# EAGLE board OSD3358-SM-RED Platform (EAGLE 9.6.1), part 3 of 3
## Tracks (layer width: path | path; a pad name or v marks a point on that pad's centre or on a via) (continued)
PMIC_PGOOD  (via drill 0.3) (continued)
  Bottom 0.152: v56.92,32.79 56.92,33.22 57.4,33.71 57.4,34.21 57.15,34.47 56.08,34.47 55.91,34.65 v55.91,35.38
PWR_BUT  (via drill 0.3)
  Top 0.152: U1.T11 57.4,35.46 v56.97,35.89 56.97,36.25 57.61,36.88 57.61,41.76 56.57,42.8 53.31,42.8 50.88,45.24 43.51,45.24 42.75,44.48 38.43,44.48 38,44.91 38,46.79 37.29,47.5 33.43,47.5 32.28,48.64 28.27,48.64 25.15,51.77 v24.18,51.77 | S2.4 12.43,51.37 12.5,51.44 | 12.5,51.44 v12.65,51.59 12.8,51.44 | S2.2 12.87,51.37 12.8,51.44 | 12.5,51.44 12.8,51.44
  Bottom 0.152: v56.97,35.89 56.44,36.42 55.68,36.42 54.56,35.31 53.09,35.31 50.95,33.17 50.95,32.89 50.57,32.51 50.57,25.04 48.54,23.01 48.54,14.58 51,12.12 51,5.56 50.37,4.93 50.37,2.97 J6.9 | v12.65,51.59 12.83,51.77 v24.18,51.77
PWR_EN  (via drill 0.3)
  Top 0.152: U1.N10 U1.N11 57.4,30.89 57.91,31.39 v57.91,31.5
  Bottom 0.152: v57.91,31.5 57.91,31.65 57.81,31.75 57.12,31.75 TP21.TP
RBIAS
  Top 0.152: U9.7 29.5,32.05 29.21,32.33 29.21,33.02 29.01,33.22 28.22,33.22 27.53,33.91 26.34,33.91 R115.1
RX_CLK
  Top 0.152: R94.1 R127.1 36.98,26.85 36.42,27.41 U9.31
RX_DV
  Top 0.152: U9.30 31.9,26.42 32.03,26.29 36.65,26.29 37.59,25.35 38.38,25.35 38.63,25.09 R101.1 R126.1
RXD0
  Top 0.152: R109.2 R125.1 36.6,25.15 35.76,25.98 31.9,25.98 31.5,26.39 U9.29
RXD1
  Top 0.152: U9.28 31.1,26.36 31.77,25.68 34.01,25.68 34.57,25.12 R106.2 R122.1
RXD2
  Top 0.152: R121.1 R98.1 32.54,25.15 32.31,25.38 30.43,25.38 30.12,25.68 30.12,26.16 30.3,26.34 U9.26
RXD3
  Top 0.152: R120.1 R95.1 30.18,24.82 30,24.99 30,25.38 29.82,25.55 29.82,26.42 29.9,26.49 U9.25
  Top 0.203: U9.25
SPI0_CS0
  Top 0.152: U18.C2 37.97,14.35 TP30.TP U21.1 39.8,14.69 39.57,14.91 R158.1
SPI0_D0(MISO)
  Top 0.152: U19.C2 38.76,12.61 TP29.TP U21.2
SPI0_D1(MOSI)
  Top 0.152: U20.C2 46.99,10.54 TP28.TP U21.5
SPI0_SCLK
  Top 0.152: U24.C2 46.33,12.41 TP27.TP U21.6
SPI1_CS0  (via drill 0.3)
  Top 0.152: U1.B1 71.32,16.89 71.6,16.61 v71.6,15.7 71.6,14.73 72.34,13.99 72.34,10.34 73.69,8.99 75.13,8.99 75.74,8.38 75.74,6.1 76.35,5.49 v77.57,5.49 | v78.72,19.43 78.72,19.81 79.5,20.6 82.53,20.6 84.73,22.81 84.73,28.19 86.72,30.18 87.96,30.18 90.55,32.76 U10.25
  Bottom 0.152: v71.6,15.7 71.96,15.7 72.26,16 77.95,16 78.72,16.76 v78.72,19.43 | J6.28 75.34,5.49 v77.57,5.49
SPI1_D0  (via drill 0.3)
  Top 0.152: v68.4,16.26 68.4,16.05 U1.A2 69.22,15.24 69.8,15.24 71.42,13.61 71.42,9.96 72.85,8.53 72.85,6.1 73.46,5.49 74.98,5.49 75.44,5.03 75.44,3.3 J6.29 | v77.95,19.43 77.95,19.76 79.1,20.9 82.4,20.9 84.43,22.94 84.43,28.32 86.59,30.48 87.83,30.48 90.05,32.69 U10.24
  Bottom 0.152: v68.4,16.26 68.1,16.56 67.67,16.56 67.41,16.31 67.41,15.93 67.79,15.54 69.6,15.54 70.36,16.31 77.83,16.31 78.41,16.89 78.41,18.47 77.95,18.92 v77.95,19.43
SPI1_D1
  Top 0.152: U1.B2 69.37,16.89 70,16.26 70.43,16.26 70.66,16.03 70.66,15.24 72.03,13.87 72.03,10.21 73.56,8.69 74.84,8.69 75.44,8.09 75.44,5.94 76.83,4.55 J6.30
SPI1_SCLK  (via drill 0.3)
  Top 0.152: v69.24,16.26 69.24,15.93 69.55,15.62 U1.A1 70.1,15.37 71.73,13.74 71.73,10.08 73.15,8.66 73.15,6.25 73.61,5.79 75.13,5.79 75.74,5.18 75.74,3.66 76.35,3.05 78.23,3.05 J6.31 | v77.19,19.43 77.19,19.74 78.66,21.21 82.27,21.21 84.12,23.06 84.12,28.45 86.46,30.79 87.68,30.79 89.55,32.65 U10.23
  Bottom 0.152: v69.24,16.26 69.6,16.61 77.7,16.61 78.11,17.02 78.11,18.06 77.19,18.97 v77.19,19.43
SYS_ADC_1P8V  (via drill 0.3)
  Top 0.152: U1.A7 62.1,15.24 62.1,13.39 v62.53,12.95 | v60.81,12.22 59.49,10.9 v57.38,10.9
  Bottom 0.152: R33.2 C10.1 57.15,11.12 v57.38,10.9 | v60.81,12.22 61.8,12.22 v62.53,12.95 63.78,14.2 72.29,14.2 72.87,14.78 73.84,14.78 74.68,13.95 74.68,12.95 79.17,8.46 79.17,4.65 J6.32
SYS_RESETN  (via drill 0.3)
  Top 0.152: U16.17 85.47,12.57 85.95,13.06 85.95,13.72 86.26,14.02 v88.24,14.02 | U1.R11 57.4,33.78 57.25,33.93 v56.74,33.93 56.19,33.93 55.37,34.75 55.37,35.69 55.93,36.25 v55.93,37.26 55.93,37.92 55.35,38.51 54.91,38.51 C94.1 R5.2 53.39,38.48 52.96,38.48 52.83,38.35 52.83,37.59 | v94.18,26.59 C14.1 95.38,26.59 95.5,26.72 95.5,29.08 95.68,29.26 96.55,29.26 96.62,29.34 97.16,29.34 97.28,29.21 101.6,29.21 102.23,29.84 J4.15 | v88.34,18.87 88.34,19.74 86.67,21.41 v86.67,22.94 | 6.44,52.95 7.53,52.95 8.18,52.3 8.18,50.93 8.61,50.49 v11.89,50.49 | v23.37,51.21 25.2,51.21 28.09,48.31 32.13,48.31 33.25,47.19 37.13,47.19 37.69,46.63 37.69,44.58 38.1,44.17 42.88,44.17 43.61,44.91 50.7,44.91 53.19,42.42 U3.4 53.19,41.76 52.88,41.45 52.5,41.45 51.82,40.77 51.82,38.48 51.36,38.02 51.36,37.54 51.69,37.21 52.45,37.21 52.7,37.47 | 52.7,37.47 52.83,37.59 | 52.83,37.59 52.96,37.47 | 52.96,37.47 53.75,36.68 TP26.P$1 | 52.7,37.47 52.96,37.47
  Top 0.254: S1.3 6.42,52.97 6.44,52.95 6.47,52.97 S1.1
  Bottom 0.152: J6.10 51.31,4.57 51.31,12.24 48.84,14.71 48.84,22.89 50.88,24.92 50.88,32.38 51.26,32.77 51.26,33.05 53.21,35 55.12,35 56.19,33.93 v56.74,33.93 | v88.24,14.02 88.24,18.77 v88.34,18.87 | v86.67,22.94 86.89,22.71 88.01,22.71 88.7,23.39 90.09,23.39 90.5,23.8 90.5,25.88 92.25,27.64 93.5,27.64 93.7,27.43 93.7,26.85 93.95,26.59 v94.18,26.59 94.74,27.15 94.74,30.2 94,30.94 91.01,30.94 90.4,31.55 86.77,31.55 84.76,29.54 83.19,29.54 83.03,29.39 83.03,28.07 82.83,27.86 80.95,27.86 80.72,28.09 77.39,28.09 76.71,28.78 76.71,30.81 76.2,31.32 74.3,31.32 71.4,28.42 69.52,28.42 69.14,28.04 67.44,28.04 66.52,28.96 64.47,28.96 63.7,29.72 63.7,32.69 62.08,34.31 58.6,34.31 57.81,35.1 57.81,36.25 56.97,37.08 56.11,37.08 v55.93,37.26 | v23.37,51.21 23.14,51.44 13.31,51.44 12.37,50.49 v11.89,50.49
SYS_RTC_1P8V  (via drill 0.3, 0.3 pad 0.61)
  Top 0.152: v52.07,37.8 52.32,38.05 52.32,39.88 TP14.TP 52.5,40.19 U3.5
  Bottom 0.152: U5.3 58.04,27 57.96,26.92 R15.1 | v56.9,27.69 57.95,27.69 U5.3 | U5.3 57.99,27.65 57.99,30.63 58.45,31.09 60.12,31.09 60.3,31.27 60.3,33.48 59.77,34.01 58.47,34.01 57.51,34.98 57.51,36.12 56.9,36.73 55.55,36.73 54.43,35.61 52.96,35.61 52.07,36.5 v52.07,37.8
  pour Top (rank 4): 56.77,26.54 56.77,28.96 58.04,28.96 58.04,26.42 56.77,26.42
  pour Bottom (no thermals): 57.63,26.14 60.17,26.14 60.38,26.34 60.38,27.97 60.2,28.14 57.66,28.14 57.48,27.97 56.77,27.97 56.64,27.84 56.64,27.28 56.87,27.05 57.23,27.05 57.48,26.8 57.48,26.29
SYS_VDD1_3P3V  (via drill 0.3, 0.3 pad 0.61, 0.5)
  Top 0.127: U7.M4 U7.N4 U7.P3 | U7.P5 77.54,40.54 v77.88,40.54 | U7.C6 U7.C7 U7.B8 U7.A9
  Top 0.152: C48.1 v19.68,11.43 R8.2 | R137.1 v33.07,12.95 | R96.1 v27.46,22.94 | R98.2 v32.54,22.94 | U16.1 80.78,15.74 80.64,15.88 v80.01,15.88 | C86.1 v91.19,12.45 | U17.D3 92.13,15.87 92.54,16.28 v93.09,16.28 | U16.8 v80.04,12.57 v80.03,12.57 | R13.2 v79.83,17.14 | 73.01,41.59 v73.13,41.71 | R44.2 R45.2 v53.37,44.93 | v57.45,45.7 R49.2 R48.2 | R130.2 v96.5,48.36 | C15.1 99.72,33.98 99.49,33.76 v99.49,33.4 | R12.2 v84.71,17.14 | R41.2 v94.18,25.53 | R144.2 v24.41,22.94 | R94.2 v39.88,25.83 | v30.5,22.94 R95.2 R93.2 | R145.1 v39.88,34.98 | Y5.4 74.13,15.76 73.89,16 72.59,16 72.49,16.1 72.49,16.94 v72.29,17.14 | R160.1 44.4,15.34 43.56,14.5 v42.55,14.5 | v37.47,16.13 37.72,15.88 U18.A2 | v37.47,13.08 37.72,12.83 U19.A2 | v47.5,8.76 47.25,9.01 U20.A2 | v47.5,11.81 47.25,12.06 U24.A2 | v38.48,9.73 39.04,9.73 39.24,9.53 R157.1 | R161.1 v37.47,8 | C85.1 86.67,14.63 v85.95,14.63 85.89,14.57 U16.22 | R40.2 v94.18,24.46 | R140.1 95.66,23.39 95.5,23.24 v95.5,22.73 | v92.2,29.84 91.39,29.84 Y3.4 | R158.2 v40.69,15.04 | U23.13 89.97,26.25 v89.97,25.2 | R5.1 53.11,39.8 52.88,39.57 v52.88,39.04 | U7.P2 U7.P1 76.99,39.12 | v69.47,43.08 69.48,43.09 U7.A9 | C87.1 v79.12,16.26
  Top 0.203: U9.3 31.1,32.12 31.47,32.49 32.18,32.49 32.64,32.94 32.64,33.5 32.84,33.71 R146.1 v33.25,32.99
  Top 0.254: U8.10 23.65,8.03 23.52,7.9 v22.91,7.9 | U8.29 27.15,14.78 27.58,15.21 v28.55,15.21 | U7.K9 74.51,43.09 | 74.51,43.09 74.49,43.09 U7.J10 | 74.51,43.09 v74.37,42.95 | U7.E6 73.01,41.59 | U7.F5 72.99,41.57 v73.13,41.71 | J4.5 v102.31,23.5 | R110.2 C39.1 v93.12,25.91 | v77.88,39.01 77.09,39.01 76.99,39.12 U7.P3 | v82.78,25.48 82.58,25.28 U22.1 82.15,25.03 U22.10 | C92.1 79.35,25.55 v79.88,25.55 79.93,25.55 80.16,25.78 U22.6
  Top 0.305: C51.1 v19.81,6.22 | U8.23 v29.72,11.43 | C93.1 v41.99,15.04 | C62.1 v22.48,8.64 | v46.35,14.35 U21.8 | v105.49,11.3 C22.1 R90.2 R89.2 R88.2 R87.2 R91.2 R86.2 v105.54,17.4 | C21.1 95.25,19.81 v93.85,19.81 | U8.15 26.15,7.25 v26.67,6.73 | C79.1 C88.1 78.66,11.68 v79.5,11.68
  Top 0.381: C63.1 v30,15.65
  Bottom 0.152: C6.2 | R84.2 R85.2 | R52.2 77.6,35.92 77.29,35.61 v76.96,35.61 | R22.2 53.87,27.79 54.13,27.53 v54.28,27.53 | C43.1 72.54,17.4 v72.29,17.14 | R92.2 v89.46,12.5 | R17.2 88.67,25.2 v89.97,25.2 | TP12.TP 62.13,22.61 v63.12,22.61
  Bottom 0.203: R146.1 v33.25,32.99
  Bottom 0.254: U6.7 U6.8 67.91,11.49 v67.56,11.15 | C6.2 v74.98,11.79 | v66.02,45.61 R46.2 R47.2 | R43.2 R42.2 v68,45.68 | R78.2 v87.61,45.54 | R79.2 v88.67,45.54 | R85.2 v95.07,45.54 | R83.2 R82.2 v91.87,45.54 | R81.2 v90.81,45.54 | R80.2 v89.74,45.54 | R76.2 R75.2 R73.2 R74.2 | R76.2 v85.47,45.54 | R77.2 R76.2 | R72.2 R71.2 R70.2 81.51,45.82 v80.37,45.82 | C20.2 C18.2 C19.2 v75.06,46.43 | R51.2 R50.2 69.98,45.68 v69.88,45.58 | C17.2 75.34,42.95 v74.37,42.95 | C90.2 89.69,23.95 89.97,24.23 v89.97,25.2
  Bottom 0.305: C16.2 v65.66,41.05 | X3.4 91.77,19.81 v93.85,19.81 | R143.2 22.55,15.67 22.99,15.24 v22.99,14.1 | v29.72,11.43 29.16,11.99 C49.1 | C50.1 v26.67,6.73
  Bottom 0.381: C76.1 v32.64,26.82
  other vias: 22.1,14.1 23.37,34.82 23.37,34.04 63.09,21.56
  pour Route15 (rank 6): -2.54,57.15 110.49,57.15 110.49,-2.54 -2.54,-2.54
  pour Top (rank 3): 61.85,21.34 64.39,21.34 64.39,23.88 61.85,23.88
  pour Top (no thermals): 20.57,14.48 20.57,13.72 20.83,13.46 22.1,13.46 22.23,13.59 23.75,13.59 23.88,13.72 23.88,14.86 23.75,14.99 21.84,14.99 21.59,14.73 20.83,14.73
  pour Bottom (no thermals): 22.99,33.78 25.15,33.78 25.15,35.05 22.99,35.05
  pour Top (no thermals): 89.71,24.97 89.71,26.39 90.27,26.39 90.27,24.97
SYS_VDD2_3P3V  (via drill 0.3, 0.3 pad 0.61)
  Top 0.152: D1.1 3.06,40.63 3.25,40.44 v13.01,40.44 | v53.11,22.55 52.81,22.25 52.81,21.77 52.53,21.49 52.07,21.49 51.92,21.64 51.56,21.64 51.36,21.44 v43.33,21.44
  Bottom 0.152: TP13.TP v56.9,22.58 56.9,23.7 56.21,24.38 54,24.38 53.47,23.85 53.47,22.91 v53.11,22.55 | v13.01,40.44 14.94,40.44 16.64,38.73 22.38,38.73 24.03,37.08 38.61,37.08 41.33,34.37 41.33,25.04 41.91,24.46 42.47,24.46 42.82,24.11 42.82,21.74 43.13,21.44 v43.33,21.44
  pour Top (rank 4): 56.77,23.88 58.04,23.88 58.04,21.34 56.77,21.34
SYS_VDD3_3P3V  (via drill 0.5)
  Bottom 0.152: TP16.TP v61.85,25.15 | v61.85,25.15 61.85,26.21 61.83,26.23 Q1.E | R20.2 R21.2 60.68,24.21 61.62,25.15 v61.85,25.15
  pour Top (rank 5): 59.94,21.34 61.21,21.34 61.21,24.51 63.12,24.51 63.12,25.78 61.21,25.78 61.21,28.96 59.94,28.96
  pour Bottom (no thermals): 59.03,23.88 60.63,23.88 61.44,24.69 62.28,24.69 62.59,24.99 62.59,26.52 62.59,26.75 61.09,26.75 61.09,25.78 61.09,25.5 61.09,25.37 61.09,25.27 61.09,25.17 60.58,24.66 59.03,24.66
SYS_VDD_1P8V  (via drill 0.3, 0.5)
  Top 0.152: U23.22 88.32,29.21 87.81,29.72 86.69,29.72 85.19,28.22 85.19,27.33 85.37,27.15 C89.1
  Top 0.254: C89.1 86.11,27.15 86.44,26.82 86.44,25.48 v86.74,25.17 86.77,25.15 87.68,25.15 87.92,25.38 U23.8
  Bottom 0.152: TP15.TP v58.04,25.15 | 86.28,26.01 R163.2 86.74,25.98 86.87,26.11 86.87,28.04 87.61,28.78 87.61,29.31 87.88,29.59 U25.2
  Bottom 0.254: 83.73,27.67 83.67,27.67 83.67,25.2 83.36,24.89 82.55,24.89 81.92,24.26 81.92,23.62 82.17,23.37 84.78,23.37 85.67,24.26 86.36,24.26 86.74,24.64 86.74,25.15 | 86.74,25.15 v86.74,25.17 | 86.28,26.01 R164.2 | 86.74,25.15 86.44,25.45 86.44,25.86 R163.2
  Bottom 0.61: v58.04,25.15 58.04,23.95 58.62,23.37 62.48,23.37 65.15,26.04 69.01,26.04 70.1,27.13 72.08,27.13 72.29,27.33 83.39,27.33 83.73,27.67 83.9,27.84 FB1.2
  pour Top (rank 5): 56.77,24.51 58.67,24.51 58.67,21.34 59.44,21.34 59.44,28.96 58.67,28.96 58.67,25.78 56.77,25.78
SYS_VOUT  (via drill 0.3, 0.5)
  Route15 0.762: v63.12,27.69 58.75,27.69 57.81,28.63 52.65,28.63 v49.4,25.38
  Bottom 0.152: TP11.TP v63.12,27.69
  Bottom 0.61: FB6.1 74.02,30.18 71.73,27.89 69.75,27.89 68.66,26.8 64.01,26.8 v63.12,27.69
  Bottom 0.762: v49.4,25.38 47.5,23.47 47.5,19.76 v45.16,17.42 45.16,9.55 48.9,5.82 J6.8 | C69.+ 34.29,18.67 35.61,17.35 v42.72,17.35
  Bottom 0.813: J6.8 J6.7
  pour Top (rank 3): 61.85,28.96 61.85,26.42 64.39,26.42 64.39,28.96
  pour Bottom (no thermals): 27.03,19.51 27.03,18.59 30.35,18.59 30.35,17.27 33.4,17.27 33.4,20.19 30.35,20.19 30.35,19.51
  pour Route15 (no thermals): 42.21,17.68 45.67,17.68 45.67,17.07 42.21,17.07
TEMP_D1+
  Top 0.152: U17.A1 93.52,14.12 94,13.64 R153.2
  Top 0.254: C84.1 R153.2
TEMP_D2+
  Top 0.152: U17.B1 93.52,14.53 94.34,15.34 95.71,15.34 95.89,15.16 C83.1
  Top 0.254: R152.2 C83.1
TEMP_D3+
  Top 0.152: U17.C1 92.95,14.91 93.47,14.91 94.23,15.67 94.23,16.28 94.49,16.54 98.2,16.54 98.45,16.28 98.45,15.54 98.3,15.39 97.1,15.39 96.9,15.19 C82.1
  Top 0.254: R151.2 C82.1
TEMP_D4+
  Top 0.152: U17.D1 92.94,15.34 93.47,15.34 93.93,15.8 93.93,16.41 94.36,16.84 98.32,16.84 98.75,16.41 98.75,15.21 98.35,14.81 C81.1
  Top 0.254: R150.2 C81.1
TEMP_D8+  (via drill 0.3)
  Top 0.152: U17.D2 92.53,15.52 92.76,15.75 93.32,15.75 93.62,16.05 93.62,16.54 93.34,16.82 v87,16.82 | C80.1 74.24,21.72 74.4,21.87 75.18,21.87 75.36,22.05 R149.2 75.77,22.35 75.89,22.23 75.89,21.16 v76.1,20.95
  Bottom 0.152: v76.1,20.95 76.15,20.9 79.3,20.9 80.54,19.66 84.81,19.66 87,17.48 v87,16.82
TEMP_D-  (via drill 0.3)
  Top 0.152: J10.3 J10.5 J10.7 J10.9 97.16,8.51 96.77,8.89 93.85,8.89 93.47,9.27 93.47,10.79 93.9,11.23 96.06,11.23 96.39,11.56 96.39,12.95 | U17.C2 U17.B2 U17.A2 | U17.A2 U17.A3 92.13,13.29 91.87,13.03 90.78,13.03 90.37,13.44 90.37,14.78 89.76,15.39 86.08,15.39 v85.24,16.23 | U17.A2 92.53,13.74 92.71,13.56 93.24,13.56 93.73,13.08 96.27,13.08 | 96.27,13.08 96.39,13.21 | 96.39,13.21 96.39,15.93 | 96.39,12.95 96.27,13.08 | C80.2 75.36,21.06 75.54,20.88 v75.54,20.42 74.55,20.42 74.27,20.7 72.62,20.7 72.47,20.85 Q2.E | 96.39,12.95 96.39,13.21
  Top 0.254: C81.2 C82.2 96.39,15.93 C83.2 C84.2
  Bottom 0.152: v75.54,20.42 76.43,20.42 76.61,20.6 79.17,20.6 80.42,19.36 84.68,19.36 85.24,18.8 v85.24,16.23
TEMP_SENSE
  Top 0.152: U1.N6 63.27,31.34 62.51,31.34 62,31.85 62,35.48 62.33,35.81 62.33,43.28 61.72,43.89 53.09,43.89 52.45,44.53 52.45,46.86 51.59,47.73 43.36,47.73 42.67,47.04 42.67,45.26 42.49,45.09 38.84,45.09 38.61,45.31 38.61,47.04 37.54,48.11 33.68,48.11 32.64,49.15 32.64,51.18 TP7.P$1
TIMER4  (via drill 0.3)
  Top 0.152: U1.M1 69.85,29.84 v69.49,29.84
  Bottom 0.152: v69.49,29.84 67.36,29.84 65.84,31.37 65.84,32.28 62.64,35.48 62.64,41.6 60.81,43.43 52.58,43.43 51.21,44.81 51.21,46.08 48.9,48.39 J5.7
TIMER5  (via drill 0.3)
  Top 0.152: U1.N3 v66.95,31.47
  Bottom 0.152: J5.9 51.44,46.74 51.84,46.33 51.84,45.09 52.88,44.04 61.37,44.04 63.25,42.16 63.25,35.74 66.95,32.03 v66.95,31.47
TIMER6  (via drill 0.3)
  Top 0.152: U1.N2 v68.22,31.47
  Bottom 0.152: v68.22,31.47 67.69,32 67.41,32 63.55,35.87 63.55,42.44 61.65,44.35 53.03,44.35 52.15,45.24 52.15,46.3 52.5,46.66 52.5,51.64 J5.10
TIMER7  (via drill 0.3)
  Top 0.152: U1.N1 69.49,31.47 v69.32,31.47
  Bottom 0.152: v69.32,31.47 69.01,31.47 68.4,30.86 68.4,30.43 68.12,30.15 67.49,30.15 66.14,31.5 66.14,32.41 62.94,35.61 62.94,41.88 61.09,43.74 52.73,43.74 51.54,44.93 51.54,46.2 49.99,47.75 49.99,51.61 J5.8
TPM_GPIO0  (via drill 0.3)
  Top 0.152: U1.F14 53.31,21.97 53.19,21.84 v53.19,21.34 | U16.12 82.47,11.71 82.75,11.43 86.28,11.43 86.44,11.58 87.17,11.58 87.63,12.04 v87.63,12.5 | v87.78,19.43 85.5,21.72 v85.5,23.24
  Bottom 0.152: v87.63,12.5 87.63,19.28 v87.78,19.43 | v53.19,21.34 53.49,21.03 66.02,21.03 66.42,20.62 67.16,20.62 67.36,20.83 67.36,23.62 70.33,26.59 76.86,26.59 77.24,26.21 77.24,24.89 77.88,24.26 80.7,24.26 81.94,23.01 85.27,23.01 v85.5,23.24
TRXN0  (via drill 0.3)
  Top 0.152: U9.10 28.3,31.87 28.09,32.08 26.85,32.08 26.64,31.88 26.64,31.57 26.34,31.27 24.92,31.27 24.31,30.66 23.67,30.66 v23.44,30.43
  Bottom 0.152: X5.3 18.3,28.84 17.86,28.4 17.17,28.4 16.84,28.73 16.84,29.59 16.99,29.74 17.42,29.74 17.58,29.9 17.58,30.38 17.4,30.56 16.99,30.56 16.84,30.71 16.84,32.13 16.66,32.31 16.66,36.14 17.5,36.98 19.15,36.98 20.07,36.07 21.13,36.07 21.74,35.46 21.74,30.99 22.07,30.66 23.22,30.66 v23.44,30.43
TRXN1  (via drill 0.3)
  Top 0.152: U9.13 27.32,30.21 27.23,30.3 26.24,30.3 26.04,30.5 25.12,30.5 24.87,30.25 24.87,29.49 24.51,29.13 23.7,29.13 v23.47,28.91
  Bottom 0.152: X5.5 18.3,32.88 17.88,32.46 17.45,32.46 17.3,32.61 17.3,35.87 17.73,36.3 18.9,36.3 19.3,35.89 19.3,29.57 19.74,29.13 20.27,29.13 20.4,29.01 20.4,28.7 20.52,28.57 20.9,28.57 21.03,28.7 21.03,29.03 21.13,29.13 23.24,29.13 v23.47,28.91
TRXN2  (via drill 0.3)
  Top 0.152: v23.47,27.38 23.7,27.61 24.94,27.61 26.34,29.01 U9.16
  Bottom 0.152: X5.8 14.75,27.86 14.25,27.36 13.89,27.36 13.74,27.51 13.74,28.75 14.2,29.21 15.29,29.21 15.75,28.75 15.75,26.85 16.28,26.31 16.87,26.31 16.97,26.21 16.97,24.61 17.73,23.85 18.92,23.85 19.61,24.54 19.61,27.25 19.99,27.64 20.34,27.64 20.5,27.48 20.5,27.13 20.62,27 21.01,27 21.13,27.13 21.13,27.51 21.26,27.64 23.22,27.64 v23.47,27.38
TRXN3  (via drill 0.3)
  Top 0.152: v23.47,25.86 23.7,26.09 25.4,26.09 27.12,27.81 U9.19
  Bottom 0.152: X5.10 14.75,33.8 14.33,33.38 13.82,33.38 12.8,32.36 12.8,26.24 14.17,24.87 15.8,24.87 17.45,23.22 19.33,23.22 20.12,24 21.67,24 22.05,24.38 22.05,25.96 22.17,26.09 23.24,26.09 v23.47,25.86
TRXP0  (via drill 0.3)
  Top 0.152: U9.9 28.7,31.91 28.22,32.38 26.72,32.38 26.34,32 26.34,31.7 26.21,31.57 24.79,31.57 24.18,30.96 23.67,30.96 v23.44,31.19
  Bottom 0.152: X5.2 18.3,27.65 17.86,28.09 17.04,28.09 16.54,28.6 16.54,32 16.36,32.18 16.36,36.27 17.37,37.29 19.28,37.29 20.19,36.37 21.26,36.37 22.05,35.59 22.05,31.11 22.2,30.96 23.22,30.96 v23.44,31.19
TRXP1  (via drill 0.3)
  Top 0.152: v23.44,29.67 23.67,29.44 24.38,29.44 24.56,29.62 24.56,30.38 24.99,30.81 26.16,30.81 26.36,30.61 U9.12
  Bottom 0.152: X5.4 18.3,31.74 17.88,32.16 17.32,32.16 16.99,32.49 16.99,35.99 17.6,36.6 19.02,36.6 19.61,36.02 19.61,29.69 19.86,29.44 23.22,29.44 v23.44,29.67
TRXP2  (via drill 0.3)
  Top 0.152: U9.15 27.3,29.41 27.23,29.34 26.24,29.34 24.82,27.91 23.7,27.91 v23.47,28.14
  Bottom 0.152: v23.47,28.14 23.27,27.94 19.86,27.94 19.3,27.38 19.3,24.66 18.8,24.16 17.86,24.16 17.27,24.74 17.27,26.34 16.99,26.62 16.41,26.62 16.05,26.98 16.05,28.88 15.42,29.52 14.07,29.52 13.44,28.88 13.44,27.38 13.77,27.05 14.25,27.05 14.75,26.55 X5.7
TRXP3  (via drill 0.3)
  Top 0.152: v23.47,26.62 23.7,26.39 25.27,26.39 27,28.12 27.25,28.12 27.35,28.21 U9.18
  Bottom 0.152: X5.9 14.75,32.65 14.33,33.07 13.95,33.07 13.11,32.23 13.11,31.14 13.28,30.96 13.66,30.96 13.82,30.81 13.82,30.35 13.69,30.23 13.26,30.23 13.11,30.07 13.11,26.36 14.3,25.17 15.93,25.17 17.58,23.52 19.2,23.52 19.99,24.31 21.54,24.31 21.74,24.51 21.74,26.09 22.05,26.39 23.24,26.39 v23.47,26.62
TX_CLK
  Top 0.152: U9.33 35.93,28.21 36.6,28.88 R135.1
TX_EN
  Top 0.152: R134.1 36.4,27.86 36.34,27.81 U9.32
TXD0
  Top 0.152: R133.1 37.19,29.9 35.9,28.61 U9.34
TXD1
  Top 0.152: U9.35 33.32,29.01 33.33,29.01 35.87,29.01 37.26,30.4 37.82,30.4 38,30.58 R132.1
TXD2
  Top 0.152: U9.36 33.3,29.41 33.34,29.36 35.79,29.36 37.47,31.04 37.47,31.29 37.59,31.42 37.82,31.42 38,31.6 R131.1
TXD3
  Top 0.152: U9.37 33.33,29.81 33.48,29.67 35.66,29.67 37.16,31.17 37.16,32.61 37.49,32.94 R129.1
UART0_RX  (via drill 0.3 pad 0.61)
  Top 0.152: U1.A12 56.57,16.05 v56.57,16.31
  Bottom 0.152: U6.6 67.92,10.49 67.74,10.31 60.58,10.31 60.27,10.62 60.27,14.43 58.4,16.31 v56.57,16.31
UART0_TX  (via drill 0.3 pad 0.61)
  Top 0.152: U1.B12 55.65,16.41 55.65,15.37 v56.11,14.91
  Bottom 0.152: U6.5 68.71,10.01 60.45,10.01 59.97,10.49 59.97,14.3 59.36,14.91 v56.11,14.91
UART1_RXD
  Top 0.152: U1.A11 57.4,14.83 56.24,13.66 56.24,10.21 55.17,9.14 55.17,6.71 55.47,6.4 66.73,6.4 67.64,5.49 70.71,5.49 J6.26
UART1_TXD
  Top 0.152: U1.B11 57.4,16.31 56.82,15.72 56.82,14.68 55.93,13.79 55.93,10.36 54.86,9.3 54.86,6.55 55.32,6.1 66.6,6.1 68.25,4.45 J6.24
UART2_RXD  (via drill 0.3)
  Top 0.152: U24.B2 46.89,12.47 46.89,11.58 47.19,11.28 48.54,11.28 R162.2 52.58,11.38 v53.98,9.98 | J6.22 65.33,5.79 55.17,5.79 54.56,6.4 54.56,7.98 53.98,8.56 v53.98,8.91
  Bottom 0.152: v53.98,9.98 v53.98,8.91
UART2_RXD_COMB
  Top 0.152: U24.A1 47.91,12.5 R162.1 53.42,12.5 54.86,13.95 U1.A13
UART2_TXD
  Top 0.152: J6.21 65.23,3.35 40.36,3.35 40.03,3.68 40.03,5.41 38.43,7.01 36.27,7.01 35.53,7.75 35.53,13.18 35.87,13.51 R156.2 36.42,13.61 37.74,13.61 38.1,13.26 38.1,12.45 U19.B2
UART2_TXD_COMB  (via drill 0.3, 0.3 pad 0.61)
  Top 0.152: U19.A1 37.05,12.39 R156.1 35.99,12.39 35.84,12.24 35.84,11.28 v36.27,10.85 | U1.B13 54.28,16.31 53.59,16.31 52.96,15.67 52.96,15.49 52.32,14.86 49.51,14.86 47.83,16.54 38.48,16.54 37.92,17.09 35.31,17.09 v34.8,16.59
  Bottom 0.152: v34.8,16.59 34.8,12.32 v36.27,10.85
UART4_RXD  (via drill 0.3)
  Top 0.152: U1.P15 52.32,32.49 52.07,32.74 v51.87,32.74
  Bottom 0.152: J6.11 52.96,1.91 52.58,2.29 52.58,5.38 51.61,6.35 51.61,12.37 49.15,14.83 49.15,22.76 51.18,24.79 51.18,32.26 51.66,32.74 v51.87,32.74
UART4_TXD  (via drill 0.3)
  Top 0.152: U1.R16 50.65,33.4 v50.39,33.15
  Bottom 0.152: J6.13 55.45,0.84 50.85,0.84 50.06,1.63 50.06,5.05 50.7,5.69 50.7,11.99 48.23,14.45 48.23,23.14 50.27,25.17 50.27,33.02 v50.39,33.15
USB0_DM  (via drill 0.3)
  Top 0.152: U1.K16 50.52,27.05 50.34,26.87 49.07,26.87 47.83,25.63 44.2,25.63 42.39,27.43 42.39,33.68 37.01,39.06 33.81,39.06 33.12,39.75 33.12,43.03 32.36,43.79 31.14,43.79 31.01,43.66 31.01,43.38 30.89,43.26 30.53,43.26 30.4,43.38 30.4,43.69 30.3,43.79 29.87,43.79 29.77,43.69 29.77,43.38 29.64,43.26 29.29,43.26 29.16,43.38 29.16,43.69 29.06,43.79 20.22,43.79 17.48,46.53 16.18,46.53 15.34,45.7 12.14,45.7 11.66,46.18 9.25,46.18 9.02,45.95 v8.64,45.95
  Bottom 0.152: X1.D- 5.07,46.03 5.21,46.18 8.03,46.18 8.26,45.95 v8.64,45.95 9.02,45.95 9.13,46.06 U2.1
USB0_DP  (via drill 0.3)
  Top 0.152: U1.K15 51.84,27.53 50.49,27.53 50.14,27.18 48.95,27.18 47.7,25.93 44.32,25.93 42.7,27.56 42.7,33.81 37.13,39.37 36.63,39.37 33.93,39.37 33.43,39.88 33.43,43.16 32.49,44.09 20.34,44.09 17.6,46.84 16.05,46.84 15.21,46 12.27,46 11.79,46.48 9.25,46.48 9.02,46.71 v8.64,46.71
  Bottom 0.152: X1.D+ 5,46.69 5.21,46.48 8.03,46.48 8.26,46.71 v8.64,46.71 9.02,46.71 9.17,46.56 U2.2
USB0_ID  (via drill 0.3)
  Top 0.152: U1.K14 53.06,27.05 52.27,27.84 50.34,27.84 49.99,27.48 48.82,27.48 47.57,26.24 44.45,26.24 43,27.69 43,33.96 40.16,36.8 v40.16,37.31
  Bottom 0.152: X1.ID 5.98,47.34 6.3,47.65 8.59,47.65 9.18,47.06 U2.3 9.64,47.31 9.88,47.55 11.4,47.55 11.84,47.12 11.84,42.65 12.9,41.58 15.09,41.58 16.03,40.64 17.78,40.64 20.07,42.93 23.27,42.93 24.31,41.88 24.31,39.09 25.4,38 39.83,38 40.16,37.67 v40.16,37.31
USB1_DM  (via drill 0.3)
  Top 0.152: U8.30 26.65,14.84 27.56,15.75 29.34,15.75 32.28,18.69 37.11,18.69 v37.34,18.47 | U1.L16 50.39,28.32 49.86,27.79 48.69,27.79 48.13,27.23 45.34,27.23 45.21,27.1 45.21,27 v45.44,26.77
  Bottom 0.152: v37.34,18.47 37.57,18.69 38.33,18.69 38.46,18.57 38.46,18.34 38.58,18.21 39.06,18.21 39.19,18.34 39.19,18.57 39.32,18.69 39.7,18.69 39.83,18.57 39.83,18.31 39.95,18.19 40.39,18.19 40.51,18.31 40.51,18.57 40.64,18.69 41.12,18.69 41.25,18.57 41.25,18.31 41.38,18.19 41.81,18.19 41.94,18.31 41.94,18.57 42.06,18.69 43.66,18.69 45.21,20.24 45.21,26.54 v45.44,26.77
USB1_DP  (via drill 0.3)
  Top 0.152: U8.31 26.15,14.78 27.43,16.05 29.18,16.05 32.13,19 37.08,19 v37.31,19.23 | U1.L15 51.84,28.8 50.44,28.8 49.73,28.09 48.56,28.09 48.01,27.53 45.19,27.53 44.88,27.23 44.88,26.98 v44.68,26.77
  Bottom 0.152: v37.31,19.23 37.54,19 43.54,19 44.91,20.37 44.91,26.54 v44.68,26.77
USB1_DRVVBUS  (via drill 0.3)
  Top 0.152: U1.M14 53.47,29.59 52.68,30.38 50.72,30.38 50.06,29.72 49.86,29.72 49.33,29.18 48.36,29.18 47.62,28.45 44.58,28.45 44.32,28.7 44.07,28.7 v43.97,28.6 | v29.34,17.75 29.34,19.76 29.64,20.07 35.03,20.07 v35.26,19.84
  Bottom 0.152: R141.2 27.99,17.27 27.72,17.54 U15.4 29.02,18.07 v29.34,17.75 | v35.26,19.84 35.48,20.07 43.74,20.07 44.3,20.62 44.3,25.43 43.84,25.88 43.84,28.47 v43.97,28.6
USB1_ID  (via drill 0.3)
  Top 0.152: U1.L14 53.24,27.96 v53.24,27.69
  Bottom 0.152: v53.24,27.69 53.24,26.11 53.72,25.63 R16.2
USB1_OCN  (via drill 0.3)
  Top 0.152: U1.R15 51.77,33.4 50.98,32.61 50.04,32.61 48.06,34.59 44.68,34.59 44.45,34.37 44.45,30.07 v43.97,29.59 | v35.23,20.6 35,20.37 27.25,20.37 v26.7,20.93
  Bottom 0.152: v35.23,20.6 35.46,20.37 43.61,20.37 43.99,20.75 43.99,25.3 43.43,25.86 43.43,29.06 v43.97,29.59 | v26.7,20.93 26.7,17.7 26.34,17.35 23.9,17.35 23.67,17.12 R143.1 23.24,16.64 23.11,16.76 23.11,18.04 U15.5
USB1_PWR
  pour Bottom (no thermals): 20.45,17.27 20.45,20.19 23.72,20.19 23.72,18.59 21.72,18.59 21.72,17.27
USB1_VBUS  (via drill 0.3)
  Top 0.152: U1.M15 51.84,30.07 50.85,30.07 50.19,29.41 49.99,29.41 49.45,28.88 48.49,28.88 47.75,28.14 44.58,28.14 v44.37,27.94
  Bottom 0.152: FB3.1 19.38,20.37 19.56,20.55 25.55,20.55 26.62,21.61 28.98,21.61 30.05,20.55 33.71,20.55 34.95,19.3 35.64,19.3 36.09,19.76 43.87,19.76 44.6,20.5 44.6,25.55 44.15,26.01 44.15,27.71 v44.37,27.94
USB_OSC1
  Top 0.152: U8.33 25.15,15.82 24.84,16.13 R108.2 C41.1 23.67,17.22 23.5,17.4 Y4.P$2
USB_OSC2
  Top 0.152: U8.32 25.65,15.82 25.96,16.13 R108.1 C40.1 27.13,17.22 27.3,17.4 Y4.P$1
USB_RESET
  Top 0.152: U8.26 28.93,12.93 28.96,12.95 R137.2 31.19,12.5 31.32,12.37 33.53,12.37 34.21,11.68 34.21,7.24 32.18,5.21 32.18,3.68 31.88,3.38 30.05,3.38 TP18.P$1
USB_UART_RX
  Top 0.152: U8.19 29.51,9.43 29.67,9.27 29.67,6.45 29.39,6.17 22.76,6.17 21.97,5.38 21.97,2.29 22.35,1.91 J9.1
USB_UART_TX
  Top 0.152: U8.21 29.5,10.43 30.28,9.65 30.28,8.91 30.45,8.74 32.72,8.74 32.99,8.46 32.99,7.75 32.66,7.42 31.06,7.42 29.52,5.87 22.89,5.87 22.35,5.33 22.35,3.43 22.61,3.17 24.77,3.17 J9.2
USBHUB0_DM  (via drill 0.3 pad 0.61)
  Top 0.152: U8.1 22.22,13.43 22.12,13.34 17.98,13.34 16.84,14.48 v16.84,16.51 17.22,16.89 U11.2
  Bottom 0.152: X5.U22 10.88,31.23 10.46,30.81 10.46,25.55 9.88,24.97 9.88,21.39 11.53,19.74 15.98,19.74 16.31,19.41 16.31,16.66 16.46,16.51 v16.84,16.51
USBHUB0_DP  (via drill 0.3 pad 0.61)
  Top 0.152: U8.2 17.8,12.93 16.28,14.45 16.28,16.82 v16.84,17.37 16.86,17.39 U11.1
  Bottom 0.152: X5.U23 11.78,30 11.58,30.2 11.1,30.2 10.77,29.87 10.77,25.4 10.19,24.82 10.19,21.54 11.68,20.04 16.15,20.04 16.64,19.56 16.64,17.58 v16.84,17.37
USBHUB1_DM  (via drill 0.3 pad 0.61)
  Top 0.152: U8.3 17.75,12.43 15.77,14.4 v15.77,18.77 16.31,19.3 U12.2
  Bottom 0.152: X5.U12 10.16,30.23 10.16,25.7 9.58,25.12 9.58,21.23 11.38,19.43 14.63,19.43 15.29,18.77 v15.77,18.77
USBHUB1_DP  (via drill 0.3 pad 0.61)
  Top 0.152: U8.4 22.18,11.93 22.1,12.01 17.6,12.01 15.21,14.4 v15.21,17.83 15.21,19 16.02,19.8 U12.1
  Bottom 0.152: X5.U13 8.18,28.25 8.18,26.31 9.27,25.22 9.27,21.08 11.23,19.13 13.92,19.13 v15.21,17.83
USBHUB2_DM  (via drill 0.3 pad 0.61)
  Top 0.152: U8.6 22.26,10.93 22.17,10.85 v16.18,10.85 15.62,10.29 U13.2
  Bottom 0.152: X4.6 12.52,10.85 v16.18,10.85
USBHUB2_DP  (via drill 0.3 pad 0.61)
  Top 0.152: U8.7 16.93,10.43 v16.5,9.99 16.12,9.62 U13.1
  Bottom 0.152: X4.7 12.52,8.84 15.84,8.84 16.5,9.49 v16.5,9.99
USBHUB3_DM  (via drill 0.3 pad 0.61)
  Top 0.152: U8.8 22.15,9.93 22.07,10.01 18.57,10.01 v18.03,9.47 U14.2
  Bottom 0.152: X4.2 10.57,10.18 10.57,9.07 11.18,8.46 17.02,8.46 v18.03,9.47
USBHUB3_DP  (via drill 0.3 pad 0.61)
  Top 0.152: U8.9 v19.15,9.43 18.83,9.43 18.53,9.14 U14.1
  Bottom 0.152: X4.3 9.2,8.53 9.65,8.08 18.41,8.08 19.15,8.81 v19.15,9.43
USR0  (via drill 0.3)
  Top 0.152: U1.P13 54.08,32.92 54.08,35 52.63,36.45 43.41,36.45 42.09,37.77 v41.99,37.77 | v10.54,49.68 10.06,50.16 3.3,50.16 3.06,49.92 D7.1
  Bottom 0.152: v10.54,49.68 12.45,47.78 12.45,42.93 13.18,42.19 15.34,42.19 16.28,41.25 17.53,41.25 19.81,43.54 23.52,43.54 24.92,42.14 24.92,39.34 25.65,38.61 40.31,38.61 41.15,37.77 v41.99,37.77
USR1  (via drill 0.3)
  Top 0.152: U1.T14 53.59,35.05 52.5,36.14 42.88,36.14 v42.01,37.01 | v10.59,48.82 9.63,49.78 4.06,49.78 3.81,49.53 3.81,47.37 3.56,47.12 D6.1
  Bottom 0.152: v42.01,37.01 41.48,37.01 40.18,38.3 25.53,38.3 24.61,39.22 24.61,42.01 23.39,43.23 19.94,43.23 17.65,40.95 16.15,40.95 15.21,41.88 13.03,41.88 12.14,42.77 12.14,47.27 v10.59,48.82
USR2  (via drill 0.3)
  Top 0.152: U1.R14 53.59,33.68 53.11,34.16 53.11,35.1 52.38,35.84 42.37,35.84 v42.01,36.2 | v10.06,40.97 8.89,42.14 8.89,43.94 8.51,44.32 3.3,44.32 3.06,44.56 D5.1
  Bottom 0.152: v10.06,40.97 14.83,40.97 16.76,39.04 22.5,39.04 24.16,37.39 38.73,37.39 39.93,36.2 v42.01,36.2
USR3  (via drill 0.3)
  Top 0.152: U1.P14 52.96,32.13 52.81,32.28 52.81,33.6 52.53,33.88 49.2,33.88 48.18,34.9 44.5,34.9 44.2,34.59 42.85,34.59 40.95,36.5 v40.95,36.78 | v8.69,41.5 7.77,42.42 3.3,42.42 3.06,42.66 D4.1
  Bottom 0.152: v40.95,36.78 39.78,36.78 38.86,37.69 24.28,37.69 22.63,39.34 16.89,39.34 14.96,41.27 10.57,41.27 10.34,41.5 v8.69,41.5
VBUS  (via drill 0.3)
  Top 0.254: U11.6 19.44,17.39 19.56,17.27 v19.56,16.66 19.94,16.66 20.07,16.79 C74.1 | U12.6 18.79,20.46 18.54,20.7 v18.03,20.7
  Bottom 0.152: R166.1 27.13,13.59 18.41,13.59
  pour Bottom: 12.83,12.83 13.46,13.46 13.46,14.61 12.83,15.24 9.4,15.24 8.89,15.75 8.89,25.02 7.75,26.16 7.75,32 8.26,32.51 12.45,32.51 13.08,33.27 13.08,34.29 12.45,34.92 7.62,34.92 7.24,34.54 7.24,25.78 8.38,24.64 8.38,15.88 7.62,15.11 7.62,13.72 8.51,12.83
  pour Top (no thermals): 18.47,8.08 18.77,8.08 18.77,6.07 18.03,5.33 13.84,5.33 13.21,5.97 13.21,12.83 12.83,13.21 8.76,13.21 8.38,13.59 8.38,14.48 8.76,14.86 12.83,14.86 13.97,13.72 13.97,6.86 14.48,6.35 15.77,6.35 16.05,6.63 16.05,8.08 16.38,8.08 16.38,6.6 16.64,6.35 18.16,6.35 18.47,6.63
  pour Bottom: 10.54,14.86 10.54,13.21 10.92,12.83 18.41,12.83 18.8,13.21 18.8,15.62 19.94,16.76 19.94,18.41 18.41,18.41 18.41,21.08 17.78,21.08 17.78,16.13 16.89,15.24 10.92,15.24
VDD_5V  (via drill 0.3, 0.5)
  Bottom 0.762: J6.6 46.35,7.01 44.25,9.12 44.25,17.98 46.58,20.32 46.58,24.03 49.53,26.98 49.53,36.88 50.16,37.52 50.16,38.3 v50.75,38.89
  Bottom 0.813: J6.6 J6.5
  other vias: 58.42,38.61 58.42,37.59 50.75,41
  pour Top (rank 3): 58.04,32 58.04,39.12 58.8,39.12 58.8,32
  pour Route15 (no thermals): 49.99,41.45 49.99,38.46 51.51,38.48 52.4,39.62 57.02,39.62 57.91,38.73 57.91,37.08 58.93,37.08 58.93,39.24 57.66,40.51 52.43,40.54 51.51,41.45
  pour Top (no thermals): 48.77,38.71 49.83,38.71 49.83,37.95 50.29,37.95 50.29,38.58 51.21,38.58 51.21,41.76 48.77,41.76 48.77,41 50.29,41 50.29,39.47 48.77,39.47
  pour Top (no thermals): 58.04,39.12 58.04,40.89 61.59,40.89 61.59,39.62 58.8,39.62 58.8,39.12
VDD_BAT  (via drill 0.5)
  Bottom 0.152: TP5.P$1 30.99,50.16 29.87,51.28 28.37,51.28 26.39,53.26 R165.2
  other vias: 60.96,38.61 60.96,37.59
  pour Top: 60.58,39.12 61.34,39.12 61.34,31.5 60.58,31.5
  pour Bottom (no thermals): 32.26,51.31 32.26,49.15 31.62,49.15 31.24,48.77 31.24,44.96 32.64,43.56 43.43,43.56 44.96,42.16 58.55,42.16 61.34,39.24 61.34,37.21 60.58,37.21 60.58,39.24 58.29,41.66 44.7,41.66 43.18,43.05 32.38,43.05 30.73,44.7 30.73,48.77 30.35,49.15 29.97,49.15 29.97,51.31
VDD_ETH_PHY  (via drill 0.3)
  Top 0.152: R124.1 24.36,33.6 23.8,33.05 v23.37,33.05 | R123.1 23.42,25.15 22.91,25.65 22.91,31.83 v23.37,32.28
  other vias: 25.93,29.82
  pour Route15 (rank 2): 13.67,24.49 16.03,24.49 16.87,23.65 16.87,21.95 21.46,21.95 21.72,21.69 21.72,21.39 21.87,21.23 23.6,21.23 23.72,21.36 23.72,23.52 24.18,23.98 25.96,23.98 26.09,24.1 26.09,25.2 28.14,27.25 28.14,31.11 27.76,31.5 27.76,33.4 27.61,33.55 22.66,33.55 22.2,34.01 22.2,38 21.69,38.51 16.87,38.51 16.87,37.34 15.37,35.84 13.56,35.84 12.65,34.92 12.65,25.5
  pour Top (no thermals): 25.12,30 28.12,30 28.12,29.62 25.12,29.62
  pour Bottom (no thermals): 25.27,32 22.99,32 22.99,33.27 25.4,33.27 25.65,33.53 25.65,34.92 26.42,34.92 26.42,33.4 26.04,33.4 25.27,32.64
VDD_HDMI_1P8V  (via drill 0.3, 0.3 pad 0.61)
  Top 0.152: U10.29 92.55,33.18 93.55,32.18 v93.55,31.47 | v95.35,38.07 v95.35,38.08
  Top 0.254: 94.11,38.08 U10.41 v95.35,38.07 | 94.11,38.08 93.73,37.69 93.73,35.92 94.26,35.38 v95.4,35.38 | U10.48 94.2,41.57 93.73,41.1 93.73,38.46 94.11,38.08 | U10.55 91.05,43.24 v91.03,43.26 | U10.5 v85.19,39.57 | U10.14 v85.19,35.07 v85.19,35.08 | C54.1 C59.1 v94.18,28.73 | v94.18,29.79 C55.1 C57.1 | C52.1 84.35,31.73 v84.61,31.47
  other vias: 83.69,31.47 83.69,30.2 95.4,42.11 95.4,41.3 84.18,30.81
  pour Route15 (no thermals): 83.21,31.62 83.21,29.95 83.52,29.64 87.4,29.64 87.99,30.23 87.99,30.56 88.65,31.22 93.78,31.22 93.78,28.17 94.61,28.17 94.61,31.04 95.86,32.28 95.86,41.99 95.22,42.62 91.47,42.62 91.47,43.69 90.53,43.69 90.53,42.67 85.6,42.67 84.96,42.04 84.96,32.38 84.51,31.93 83.52,31.93
  pour Bottom (no thermals): 82.45,31.75 82.45,29.69 82.5,29.64 85.24,29.67 85.24,31.6 84.96,31.93 84.79,31.93 84.79,32.61 83.9,32.61 83.9,31.93 82.78,31.93
  pour Top (no thermals): 94.26,42.42 94.26,40.46 95.35,40.46 95.35,40.69 95.89,41.22 95.89,42.42
  pour Top (no thermals): 94.26,35.79 94.26,34.98 95.89,34.98 95.89,35.79
VDD_USB_5V  (via drill 0.3, 0.3 pad 0.61, 0.5)
  Top 0.152: U1.J16 50.72,25.78 49.66,24.71 43.81,24.71 43.26,25.27 42.52,25.27 v42.29,25.5
  Top 0.254: v11.1,45.64 11.63,45.64 11.94,45.34 12.62,45.34 13.39,44.58 v14.22,44.58 | C3.1 12.95,41.73 12.95,42.8
  Bottom 0.152: U2.6 10.38,45.81 10.54,45.64 v11.1,45.64 | v42.29,25.5 42.67,25.88 42.67,37.97 38.35,42.29
  other vias: 59.69,38.61 59.69,37.59 14.22,43.81 14.22,43.05
  pour Top (rank 2): 59.31,39.12 60.07,39.12 60.07,31.5 59.31,31.5
  pour Bottom (no thermals): 13.34,44.96 14.48,44.96 14.73,45.21 14.73,48.64 15.62,49.53 25.15,49.53 26.16,48.51 26.16,44.32 27.94,42.55 42.93,42.55 45.19,40.41 58.78,40.41 60.07,39.12 60.07,37.21 59.31,37.21 59.31,39.12 58.55,39.9 44.96,39.9 42.67,42.04 27.69,42.04 25.65,44.2 25.65,48.26 24.89,49.02 15.75,49.02 15.24,48.51 15.24,43.05 14.86,42.67 13.34,42.67
  pour Top (no thermals): 14.86,44.96 14.86,42.67 12.95,42.67 12.95,44.96
VIN  (via drill 0.3)
  Top 0.152: U4.2 48.39,37.72 48.66,37.45 U4.4 48.27,36.83 43.64,36.83 42.67,37.8 v42.67,38.86
  Bottom 0.152: R6.2 42.93,39.12 v42.67,38.86
  pour Top (no thermals): 34.16,39.75 37.34,39.75 38.61,38.48 42.93,38.48 43.43,39.12 45.72,39.12 45.72,40.13 43.81,40.13 43.81,41.02 45.72,41.02 45.72,41.66 39.24,41.66 36.96,43.94 34.29,43.94 33.78,43.43 33.78,40.13
VIN_CTL  (via drill 0.3 pad 0.61)
  Top 0.152: U26.2 46.54,40.58 47.09,40.03 v47.09,39.17
  Bottom 0.152: 47.02,37.06 R167.2 47.09,37.08 v47.09,39.17 45.44,39.17 R6.1
VIN_PREDIODE  (via drill 0.3)
  other vias: 19.56,41.53 23.75,41.53 23.75,40.64 23.75,39.88 19.56,40.64 19.56,39.88
  pour Top: 19.56,39.12 32.64,39.12 32.64,41.78 28.7,41.78 27.81,42.67 19.56,42.67 18.8,41.91 18.8,39.88
  pour Bottom: 18.92,42.67 18.92,39.5 24.13,39.5 24.13,42.67
VIN_PREFUSE
  pour Top (no thermals): 28.19,47.88 28.19,44.7 36.96,44.7 36.96,46.74 33.15,46.74 32,47.88
VREF2
  Bottom 0.152: U25.8 U25.7 90.12,29.59 90.19,29.59 90.63,29.16 90.63,26.47 89.89,25.73 87.63,25.73 87.5,25.6 R17.1
VREFN  (via drill 0.3)
  Top 0.152: U1.B9 59.94,16.84 59.46,16.36 59.46,14.38 v59.23,14.15
  Bottom 0.152: R25.1 v59.23,14.15
VREFP  (via drill 0.3)
  Top 0.152: U1.B7 62.03,16.43 v61.92,16.43
  Bottom 0.152: R33.1 C9.1 C8.1 54.1,14.94 56.69,17.53 60.83,17.53 v61.92,16.43
XDMA_EVENT_INTR0  (via drill 0.3)
  Top 0.152: v70.1,9.02 69.83,9.3 67.44,9.3 67.22,9.51 C1.2 67.22,10.71 66.93,11 66.93,11.3 67.37,11.75 67.37,12.59 R4.2 | v78.64,7.01 79.1,7.01 79.55,6.55 97.84,6.55 98.45,7.16 98.45,7.85 100.66,10.06 105.79,10.06 106.17,10.44 106.17,30.73 105.79,31.11 J4.17
  Bottom 0.152: v70.1,9.02 70.56,8.56 70.56,7.04 71.2,6.4 75.06,6.4 75.74,7.09 75.74,8.38 76.05,8.69 78.33,8.69 78.64,8.38 v78.64,7.01

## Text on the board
tPlace: 2 | 46 | SEE | RST | PWR | 45 | BACK | BAT | BOOT | OSD3358-512M-BSM | OSD335x-SM | EVALUATION BOARD | Rev 4 | DCAN | 46 | 1 | 45
bPlace: GND | PMIC_TS | BAT_SENSE | VIN_BAT
tNames: RX | TX | RX | TX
